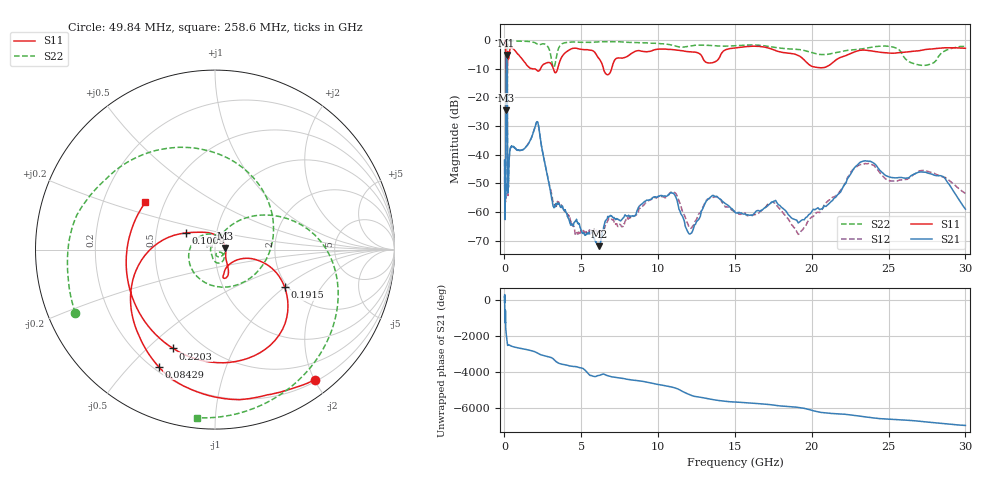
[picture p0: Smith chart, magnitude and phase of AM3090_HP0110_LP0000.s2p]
! Date/Time: Thu, Feb 28, 2019 1:59 PM
! Network Analyzer: Agilent Technologies E8364B Rev: A.07.50.67
! Sweep from 0.010 to 30.000 GHz, 1601 Points, Sweep Type: LOG
! Power Supply: 5.023 V, 0.002 A
# Hz S DB R 50
!freq MagS11 AngS11 MagS21 AngS21 MagS12 AngS12 MagS22 AngS22
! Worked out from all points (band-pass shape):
!   1601 points, 10 MHz to 30 GHz, reference 50 ohm
!   highest |S21| = -5.22 dB at 139 MHz (marker M1); lowest = -71.9 dB at 6.171 GHz (marker M2)
!   |S21| within 3 dB of the highest: 108.7 MHz to 175.4 MHz (66.66 MHz wide, 46.9 % of centre)
!   lowest |S11| = -24.6 dB at 107.7 MHz (marker M3), VSWR 1.13, Z = 56.2 + j1.1 ohm
!   |S11| at or under -10 dB: 1.94 GHz to 2.349 GHz (409.4 MHz wide, 19.1 % of centre); 3.183 GHz to 3.464 GHz (281.5 MHz wide, 8.47 % of centre); 6.447 GHz to 6.977 GHz (529.5 MHz wide, 7.89 % of centre)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
!   |S22| runs from -33.3 to -0.1 dB; largest |S21 - S12| = 0.012
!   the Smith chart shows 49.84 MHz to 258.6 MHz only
!   S11 on the Smith chart (normalised r, x): 49.84 MHz: 0.23, -2.01; 84.29 MHz: 0.22, -0.61; 100.9 MHz: 0.71, +0.14; 191.5 MHz: 1.93, -0.99; 220.3 MHz: 0.35, -0.60; 258.6 MHz: 0.39, +0.26
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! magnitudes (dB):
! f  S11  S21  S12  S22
! 10 MHz  -0.3  -41.8  -42.0  -0.5
! 38.04 MHz  -0.5  -59.6  -58.4  -1.2
! 49.84 MHz  -0.8  -51.9  -49.4  -1.4
! 84.29 MHz  -2.8  -48.4  -47.6  -6.0
! 100.9 MHz  -14.6  -14.5  -14.6  -15.2
! 107.7 MHz  -24.6  -8.7  -8.7  -19.3
! 139 MHz  -16.5  -5.2  -5.2  -32.4
! 144.7 MHz  -16.9  -5.3  -5.2  -25.9
! 171.5 MHz  -16.5  -7.3  -7.3  -31.6
! 191.5 MHz  -7.1  -22.4  -22.2  -8.5
! 220.3 MHz  -4.5  -53.4  -53.8  -1.3
! 258.6 MHz  -6.6  -50.8  -49.1  -0.5
! 550.5 MHz  -3.0  -37.2  -37.4  -0.2
! 2.084 GHz  -10.5  -28.7  -28.7  -1.3
! 3.253 GHz  -11.1  -58.3  -57.5  -9.2
! 6.171 GHz  -6.6  -71.9  -67.7  -0.6
! 7.926 GHz  -5.9  -61.4  -62.6  -0.8
! 10.81 GHz  -3.3  -53.3  -53.2  -1.7
! 12.13 GHz  -4.1  -67.5  -65.7  -2.1
! 19.31 GHz  -6.0  -62.9  -66.6  -3.4
! 23.59 GHz  -3.6  -42.2  -43.2  -2.8
! 30 GHz  -2.9  -59.0  -53.5  -2.2
